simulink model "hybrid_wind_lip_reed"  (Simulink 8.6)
settings: Solver=FixedStepDiscrete  SolverMode=SingleTasking  StartTime=0.0  StopTime=inf  FixedStep=Ts  RelTol=1e-3
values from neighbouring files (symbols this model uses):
  ae = 1.5 gives smoother results, so more realistic, but it destabilises the hybrid instrument!    [lip_reed.m]
  alpha_Qr = alpha_wr/alpha_r    [lip_reed.m]
  alpha_wr = sqrt(alpha_k)    [lip_reed.m]
  amp_gain_factor = 0.73316    [hybrid_wind.m]    (also in measurements.m = 0.73312)
  gammal_cte = 2    [lip_reed.m]
  HLL_d = c2d(HLL_c,Ts)    [hybrid_wind.m]    (also in measurements.m)
  maxoutputvoltage = 5    [hybrid_wind.m]    (also in measurements.m)
  micoffset_V = mean(voltsin_calib)    [hybrid_wind.m]    (also in measurements.m)
  micpreampsensitivity = -0.0025726    [hybrid_wind.m]    (also in measurements.m)
  PM = 50    [bowed_string_hyperbolic.m]    (also in lip_reed.m = 20; single_reed.m = 100)
  Qr = 3    [lip_reed.m]    (also in single_reed.m = 5)
  Ts = 25e-6    (= 2.5e-05)    [hybrid_wind.m]    (also in measurements.m)
  wr = 2*pi*140*0.7    (= 615.752160104)    [lip_reed.m]    (also in single_reed.m = 15707.9632679)
  yb = 1    [lip_reed.m]
  yth = yb+0.2    (= 1.2)    [lip_reed.m]
  Zc = rho*c/St    (= 2615281.00417)    [hybrid_wind.m]
  zetal = 0.15    [lip_reed.m]
undefined symbols (not defined in the file or in its folder): Bl, cell2mat, Mms, Re, Sd, sigbuilder_block, vibrato
libraries: simulink x3

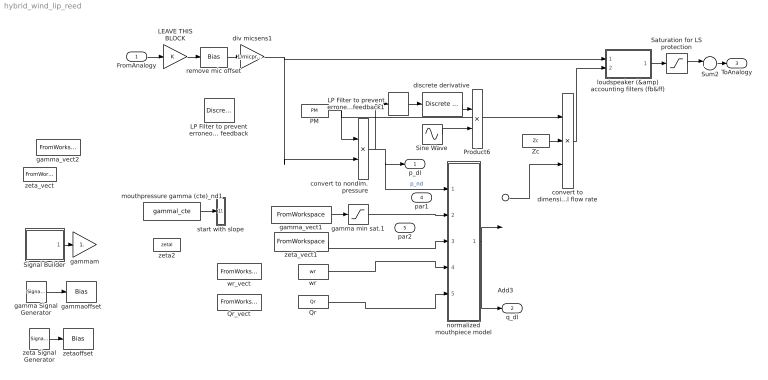
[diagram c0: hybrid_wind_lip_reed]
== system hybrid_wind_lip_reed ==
  FromAnalogy : Inport
  Add3 : Sum
  LEAVE THIS BLOCK : Gain
  LP Filter to prevent erroneous high freq feedback : DiscreteFilter  Numerator=HdLP.ScaleValues(1)*HdLP.sosMatrix(1:end/2)  Denominator=HdLP.ScaleValues(2)*HdLP.sosMatrix(1+end/2:end)  SampleTime=Ts
  LP Filter to prevent erroneous high freq feedback1 : DiscreteFilter  Numerator=HdLP2.ScaleValues(1)*HdLP2.sosMatrix(1:end/2)  Denominator=HdLP2.ScaleValues(2)*HdLP2.sosMatrix(1+end/2:end)  SampleTime=Ts
  PM : Constant  Value=PM
  Product6 : Product
  Qr : Constant  Value=Qr
  Qr_vect : FromWorkspace  VariableName=Qr_vect  SampleTime=0  OutputAfterFinalValue=Setting to zero
  Saturation for LS protection : Saturate  UpperLimit=maxoutputvoltage  LowerLimit=-maxoutputvoltage
  Signal Builder : Subsystem  Tag=STV Subsys  LoadFcn=sigbuilder_block('load');  StartFcn=sigbuilder_block('start');  StopFcn=sigbuilder_block('stop');  ClipboardFcn=sigbuilder_block('clipboard');
  Sine Wave : Sin  Amplitude=vibrato.amp  Bias=-vibrato.amp  Frequency=vibrato.freq*2*pi  SampleTime=0
  Sum2 : Sum  Inputs=|++
  Zc : Constant  Value=Zc
  convert to dimensional flow rate : Product  Inputs=*/*
  convert to nondim. pressure : Product  Inputs=/*
  discrete derivative : simulink/Discrete/Discrete Derivative  gainval=1.0  ICPrevScaledInput=0.0  InputProcessing=Inherited  OutMin=[]  OutMax=[]  OutDataType=fixdt(1, 16)  OutScaling=2^-10  DoSatur=off
  div micsens1 : Gain  Gain=1/micpreampsensitivity
  gamma Signal Generator : SignalGenerator  WaveForm=sawtooth  Amplitude=(3-1)/2  Frequency=0.2
  gamma min sat.1 : Saturate  UpperLimit=100  LowerLimit=0.3
  gamma_vect1 : FromWorkspace  VariableName=gammal_envs_all  SampleTime=0
  gamma_vect2 : FromWorkspace  VariableName=gammal_vect  SampleTime=0  OutputAfterFinalValue=Setting to zero
  gammam : Gain  Gain=1.
  gammaoffset : Bias  Bias=0.4+(0.9-0.4)/2
  loudspeaker (&amp) accounting filters (fb&ff) : Subsystem
  mouthpressure gamma (cte)_nd1 : Constant  Value=gammal_cte
  normalized mouthpiece model : Subsystem
  remove mic offset : Bias  Bias=-micoffset_V
  start with slope : Subsystem
  wr : Constant  Value=wr
  wr_vect : FromWorkspace  VariableName=wr_vect  SampleTime=0  OutputAfterFinalValue=Setting to zero
  zeta Signal Generator : SignalGenerator  WaveForm=sawtooth  Amplitude=(0.3-0.1)/2  Frequency=10
  zeta2 : Constant  Value=zetal
  zeta_vect : FromWorkspace  VariableName=zetal_vect  SampleTime=0  OutputAfterFinalValue=Setting to zero
  zeta_vect1 : FromWorkspace  VariableName=zetal_envs_all  SampleTime=0  OutputAfterFinalValue=Setting to zero
  zetaoffset : Bias  Bias=0.1+(0.3-0.1)/2
  p_dl : Outport
  q_dl : Outport  Port=2
  ToAnalogy : Outport  Port=3
  par1 : Outport  Port=4
  par2 : Outport  Port=5
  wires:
  Saturation for LS protection/1 -> Sum2/1
  FromAnalogy/1 -> LEAVE THIS BLOCK/1
  loudspeaker (&amp) accounting filters (fb&ff)/1(V_amp_in) -> Saturation for LS protection/1
  normalized mouthpiece model/1(u_nd) -> Add3/2, q_dl/1
  PM/1 -> convert to nondim. pressure/1, convert to dimensional flow rate/1
  Zc/1 -> convert to dimensional flow rate/2
  convert to nondim. pressure/1 -> p_dl/1, normalized mouthpiece model/1(p), LP Filter to prevent erroneous high freq feedback1/1  "p_nd"
  Sum2/1 -> ToAnalogy/1
  div micsens1/1 -> loudspeaker (&amp) accounting filters (fb&ff)/1(P), convert to nondim. pressure/2
  zeta Signal Generator/1 -> zetaoffset/1
  gamma Signal Generator/1 -> gammaoffset/1
  Signal Builder/1(Signal 1) -> gammam/1
  discrete derivative/1 -> Product6/1
  Sine Wave/1 -> Product6/2
  convert to dimensional flow rate/1 -> loudspeaker (&amp) accounting filters (fb&ff)/2(U_calc)
  Add3/1 -> convert to dimensional flow rate/3
  LP Filter to prevent erroneous high freq feedback1/1 -> discrete derivative/1
  mouthpressure gamma (cte)_nd1/1 -> start with slope/1(gamma_in)
  gamma min sat.1/1 -> normalized mouthpiece model/2(gamma)
  Qr/1 -> normalized mouthpiece model/5(Qr)
  wr/1 -> normalized mouthpiece model/4(wr)
  remove mic offset/1 -> div micsens1/1
  LEAVE THIS BLOCK/1 -> remove mic offset/1
  gamma_vect1/1 -> gamma min sat.1/1
  zeta_vect1/1 -> normalized mouthpiece model/3(zeta)

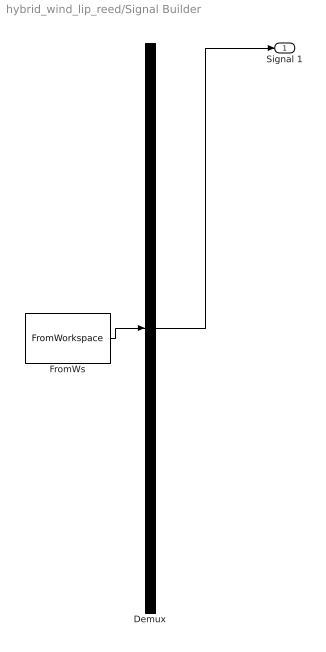
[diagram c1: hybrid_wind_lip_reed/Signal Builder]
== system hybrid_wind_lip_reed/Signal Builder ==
  Demux : Demux  Tag=STV Demux  Outputs=1
  FromWs : FromWorkspace  Tag=STV FromWs  VariableName=tuvar  SampleTime=0  SigBuilderData=DataTag0  VnvData=DataTag1
  Signal 1 : Outport  Tag=STV Outport
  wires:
  Demux/1 -> Signal 1/1
  FromWs/1 -> Demux/1

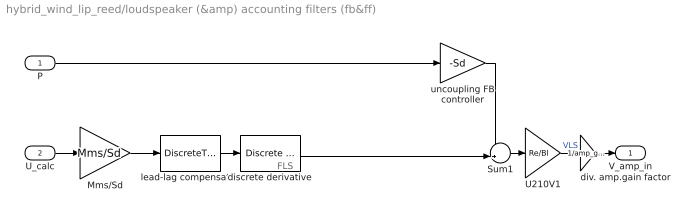
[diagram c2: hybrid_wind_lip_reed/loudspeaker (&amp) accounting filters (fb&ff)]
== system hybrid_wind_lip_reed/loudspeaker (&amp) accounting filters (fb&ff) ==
  note: FLS
  P : Inport
  U_calc : Inport  Port=2
  Mms/Sd : Gain  Gain=Mms/Sd
  Sum1 : Sum  Inputs=-+|
  U210V1 : Gain  Gain=Re/Bl
  discrete derivative : simulink/Discrete/Discrete Derivative  gainval=1.0  ICPrevScaledInput=0.0  InputProcessing=Inherited  OutMin=[]  OutMax=[]  OutDataType=fixdt(1, 16)  OutScaling=2^-10  DoSatur=off
  div. amp.gain factor : Gain  Gain=1/amp_gain_factor
  lead-lag compensator : DiscreteTransferFcn  Numerator=cell2mat(HLL_d.num)  Denominator=cell2mat(HLL_d.den)  SampleTime=Ts
  uncoupling FB controller : Gain  Gain=-Sd
  V_amp_in : Outport
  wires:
  Sum1/1 -> U210V1/1
  U210V1/1 -> div. amp.gain factor/1  "VLS"
  U_calc/1 -> Mms/Sd/1
  discrete derivative/1 -> Sum1/2
  uncoupling FB controller/1 -> Sum1/1
  div. amp.gain factor/1 -> V_amp_in/1
  P/1 -> uncoupling FB controller/1
  Mms/Sd/1 -> lead-lag compensator/1
  lead-lag compensator/1 -> discrete derivative/1

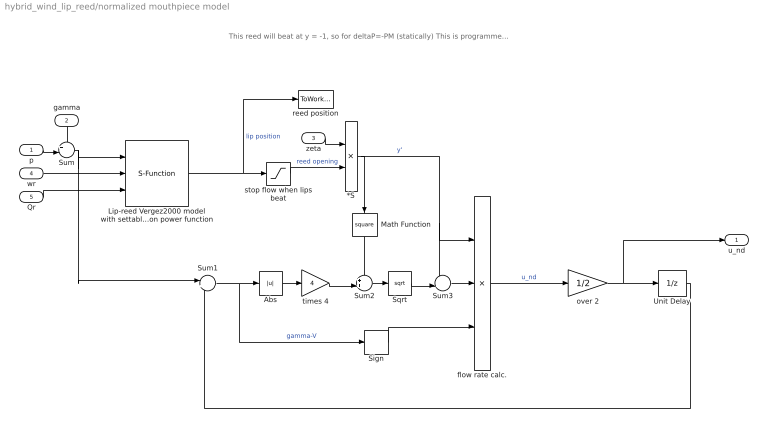
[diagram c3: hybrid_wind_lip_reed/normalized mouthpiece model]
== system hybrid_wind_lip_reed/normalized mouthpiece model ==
  note: This reed will beat at y = -1, so for deltaP=-PM (statically) This is programmed in the LP filter, which switches coefficients.
  p : Inport
  gamma : Inport  Port=2
  zeta : Inport  Port=3
  wr : Inport  Port=4
  Qr : Inport  Port=5
  *S : Product  Inputs=**
  Abs : Abs
  Lip-reed Vergez2000 model with settable rest-position offset and opening section power function : S-Function  InitFcn=try, set_param(gcb,'FunctionName','reed_discrete_LP_filter_hitting_reed'), end  FunctionName=reed_discrete_LP_filter_hitting_reed  Parameters=1/Ts,alpha_wr,alpha_Qr,yth,yb,ae  SFunctionModules=reed_discrete_LP_filter_hitting_reed_wrapper  WizardData=DataTag2  SFunctionDeploymentMode=off  EnableBusSupport=off
  Math Function : Math  Operator=square
  Sign : Signum
  Sqrt : Sqrt
  Sum : Sum  Inputs=+-|
  Sum1 : Sum  Inputs=|++
  Sum2 : Sum  Inputs=++|
  Sum3 : Sum  Inputs=-+|
  Unit Delay : UnitDelay  SampleTime=-1
  flow rate calc. : Product  Inputs=3
  over 2 : Gain  Gain=1/2
  reed position : ToWorkspace  VariableName=y_dl  SaveFormat=Structure  SampleTime=-1
  stop flow when lips beat : Saturate  UpperLimit=100  LowerLimit=0
  times 4 : Gain  Gain=4
  u_nd : Outport
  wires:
  p/1 -> Sum/2
  zeta/1 -> *S/1
  Sum2/1 -> Sqrt/1
  Sum1/1 -> Abs/1, Sign/1  "gamma-V"
  Sum/1 -> Sum1/1, Lip-reed Vergez2000 model with settable rest-position offset and opening section power function/1
  *S/1 -> flow rate calc./1, Sum3/1, Math Function/1  "y'"
  flow rate calc./1 -> over 2/1  "u_nd"
  Sqrt/1 -> Sum3/2
  Sum3/1 -> flow rate calc./2
  over 2/1 -> u_nd/1, Unit Delay/1
  Math Function/1 -> Sum2/1
  Abs/1 -> times 4/1
  times 4/1 -> Sum2/2
  Sign/1 -> flow rate calc./3
  Unit Delay/1 -> Sum1/2
  wr/1 -> Lip-reed Vergez2000 model with settable rest-position offset and opening section power function/2
  Qr/1 -> Lip-reed Vergez2000 model with settable rest-position offset and opening section power function/3
  stop flow when lips beat/1 -> *S/2  "reed opening"
  Lip-reed Vergez2000 model with settable rest-position offset and opening section power function/1 -> stop flow when lips beat/1, reed position/1  "lip position"
  gamma/1 -> Sum/1

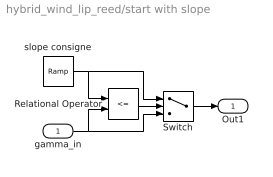
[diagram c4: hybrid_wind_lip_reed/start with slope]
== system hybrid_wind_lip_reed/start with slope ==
  gamma_in : Inport
  Relational Operator : RelationalOperator  Operator=<=  OutDataTypeStr=boolean
  Switch : Switch  Criteria=u2 > Threshold
  slope consigne : simulink/Sources/Ramp  slope=gammal_cte*100  start=0  X0=0
  Out1 : Outport
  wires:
  slope consigne/1 -> Relational Operator/1, Switch/1
  gamma_in/1 -> Relational Operator/2, Switch/3
  Relational Operator/1 -> Switch/2
  Switch/1 -> Out1/1
